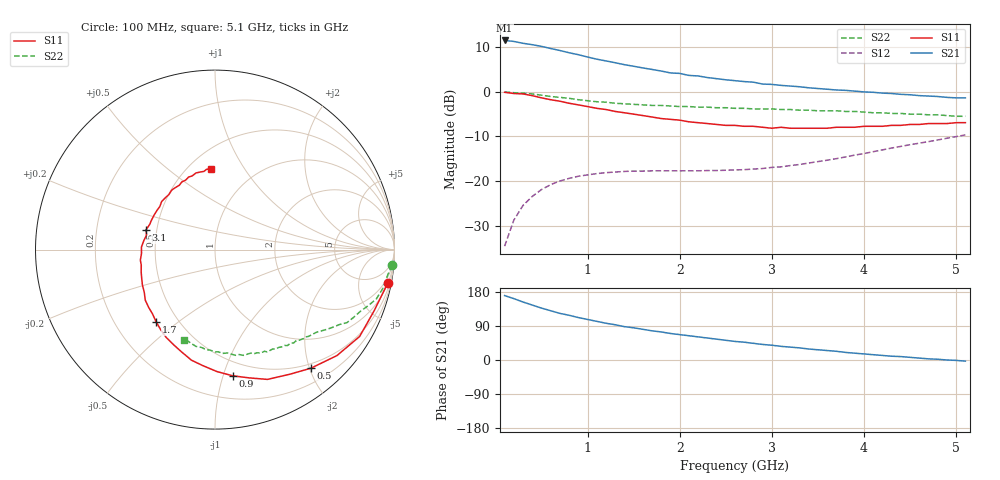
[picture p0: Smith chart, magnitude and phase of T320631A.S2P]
!AT-32063
!S AND NOISE PARAMETERS per side at Vce=1.0 V  Ic=1mA.  LAST UPDATED 11-11-96
# ghz s ma r 50
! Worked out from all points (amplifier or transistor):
!   51 points, 100 MHz to 5.1 GHz, reference 50 ohm
!   highest |S21| = 11.4 dB at 100 MHz (marker M1)
!   |S21| within 3 dB of that: start of sweep to 861.4 MHz
!   unconditionally stable (mu >= 1): 1.994 GHz to end of sweep
!   at 900 MHz: K = 0.46, MSG = 13.5 dB, |S12| = -18.9 dB
!   at 2.6 GHz: K = 1.26, MAG = 6.9 dB, |S12| = -17.5 dB
!   at 5.1 GHz: K = 1.01, MAG = 3.5 dB, |S12| = -9.7 dB
!   lowest NFmin = 0.71 dB at 9 GHz
!   S11 on the Smith chart (normalised r, x): 100 MHz: 1, -10; 500 MHz: 0.43, -2.02; 900 MHz: 0.38, -1.08; 1.7 GHz: 0.38, -0.42; 3.1 GHz: 0.44, +0.11; 5.1 GHz: 0.64, +0.72
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0.1  0.98 -11.0  3.7 170.0  0.019 83.0  0.99 -5.0
0.2  0.95 -21.0  3.61 162.0  0.037 77.0  0.97 -9.0
0.3  0.94 -31.0  3.44 153.0  0.054 70.0  0.96 -13.0
0.4  0.9 -41.0  3.32 145.0  0.068 65.0  0.94 -17.0
0.5  0.85 -51.0  3.18 137.0  0.081 59.0  0.91 -20.0
0.6  0.81 -59.0  3.01 130.0  0.092 54.0  0.88 -23.0
0.7  0.78 -68.0  2.86 123.0  0.101 50.0  0.86 -26.0
0.9  0.71 -82.0  2.57 112.0  0.114 43.0  0.81 -31.0
1  0.68 -89.0  2.42 107.0  0.118 40.0  0.79 -33.0
1.2  0.63 -102.0  2.19 97.0  0.125 35.0  0.76 -36.0
1.4  0.58 -113.0  1.99 88.0  0.129 32.0  0.73 -39.0
1.7  0.52 -129.0  1.76 77.0  0.131 29.0  0.7 -44.0
1.8  0.5 -134.0  1.69 74.0  0.131 28.0  0.7 -45.0
1.9  0.49 -139.0  1.61 70.0  0.131 27.0  0.69 -47.0
2  0.48 -144.0  1.59 67.0  0.131 28.0  0.68 -48.0
2.1  0.46 -149.0  1.51 64.0  0.131 28.0  0.68 -50.0
2.2  0.45 -154.0  1.49 61.0  0.131 28.0  0.67 -51.0
2.6  0.42 -172.0  1.32 49.0  0.134 31.0  0.65 -57.0
3.1  0.4 164.0  1.17 36.0  0.145 37.0  0.63 -64.0
3.5  0.39 146.0  1.08 27.0  0.166 41.0  0.61 -71.0
4.3  0.42 116.0  0.95 10.0  0.235 43.0  0.57 -88.0
5.1  0.45 93.0  0.85 -3.0  0.329 37.0  0.53 -109.0
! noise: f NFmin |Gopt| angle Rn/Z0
9  0.71  0.76  50  0.44
1.8  1.37  0.6  112  0.24
2.4  1.8  0.5  155  0.1
